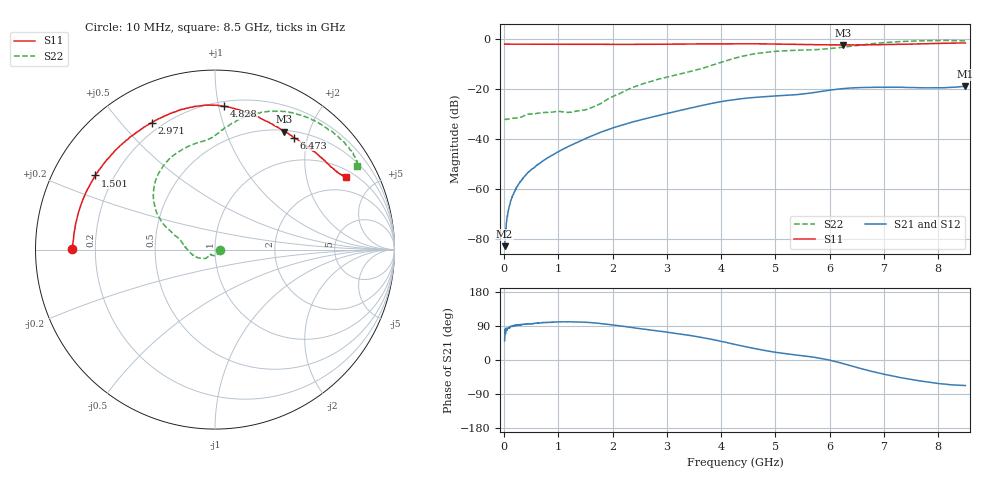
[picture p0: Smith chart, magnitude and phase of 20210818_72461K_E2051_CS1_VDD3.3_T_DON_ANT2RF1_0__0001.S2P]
!Agilent Technologies,E5071C,MY46417908,A.11.23
!Date: Wed Aug 18 14:23:53 2021
!Data & Calibration Information:
!Freq	S11:SOLT2(ON)	S21:SOLT2(ON)	S12:SOLT2(ON)	S22:SOLT2(ON)
!PortZ  Port1:50+j0  Port2:50+j0
!Above PortZ is port z conversion or system Z0 setting when saving the data.
!When reading, reference impedance value at option line is always used.
# Hz S dB R 50
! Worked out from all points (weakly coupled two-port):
!   1601 points, 10 MHz to 8.5 GHz, reference 50 ohm
!   highest |S21| = -18.94 dB at 8.5 GHz (marker M1); lowest = -82.9 dB at 10 MHz (marker M2)
!   lowest |S11| = -2.4 dB at 6.25 GHz (marker M3), VSWR 7.38, Z = 25.9 + j81 ohm
!   |S11| at or under -10 dB: nowhere
!   |S22| runs from -32.2 to -0.5 dB; largest |S21 - S12| = 0.00051
!   S11 on the Smith chart (normalised r, x): 10 MHz: 0.11, +0.00; 1.501 GHz: 0.13, +0.28; 2.971 GHz: 0.16, +0.61; 4.828 GHz: 0.23, +1.04; 6.473 GHz: 0.59, +1.77; 8.5 GHz: 1.29, +3.41
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1e7  -1.98 179.7  -82.92 50.5  -81.90 71.1  -31.93 -3.0
8.42875e7  -2.02 178.2  -68.27 85.8  -68.49 86.5  -31.97 -14.2
1.320438e8  -2.02 177.2  -64.19 89.8  -64.36 86.3  -31.78 -20.4
2.169438e8  -2.04 175.4  -59.87 90.7  -60.15 91.6  -31.63 -32.4
3.442938e8  -2.05 172.7  -55.76 94.2  -55.85 93.7  -30.95 -55.0
4.716438e8  -2.05 170.1  -52.86 95.5  -52.84 95.3  -29.98 -71.3
7.741e8  -2.07 163.6  -47.99 98.8  -47.96 99.3  -29.35 -103.2
1.426769e9  -2.11 149.8  -40.55 100.0  -40.54 100.0  -28.60 -131.1
1.501056e9  -2.12 148.2  -39.82 99.6  -39.83 99.6  -28.30 -130.3
2.328831e9  -2.12 130.1  -33.43 86.4  -33.43 86.4  -19.72 -153.7
2.843538e9  -2.06 119.1  -30.61 76.5  -30.62 76.4  -16.04 178.5
2.970888e9  -2.05 116.5  -29.94 74.0  -29.93 74.0  -15.35 173.4
3.809275e9  -1.90 101.7  -25.83 55.0  -25.84 55.0  -10.63 155.7
4.255e9  -1.87 94.7  -24.18 41.1  -24.19 41.1  -7.64 144.1
4.828075e9  -1.94 86.4  -23.01 24.6  -23.02 24.6  -5.27 122.3
5.23135e9  -2.06 79.7  -22.51 15.7  -22.51 15.7  -4.61 107.3
5.671769e9  -2.20 71.8  -21.53 8.1  -21.53 8.2  -4.28 95.0
6.25015e9  -2.37 59.7  -19.82 -9.7  -19.83 -9.7  -3.24 84.3
6.473012e9  -2.36 55.0  -19.51 -18.6  -19.52 -18.6  -2.62 79.1
7.088538e9  -2.15 42.3  -19.28 -40.2  -19.32 -40.3  -1.26 62.6
7.926925e9  -1.74 30.8  -19.52 -60.4  -19.50 -60.5  -0.58 40.0
8.5e9  -1.58 29.0  -18.94 -67.4  -18.95 -67.6  -0.76 30.4
